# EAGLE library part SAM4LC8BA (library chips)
SAM4L Microcontroller. 64QFN Package. 512 Flash.
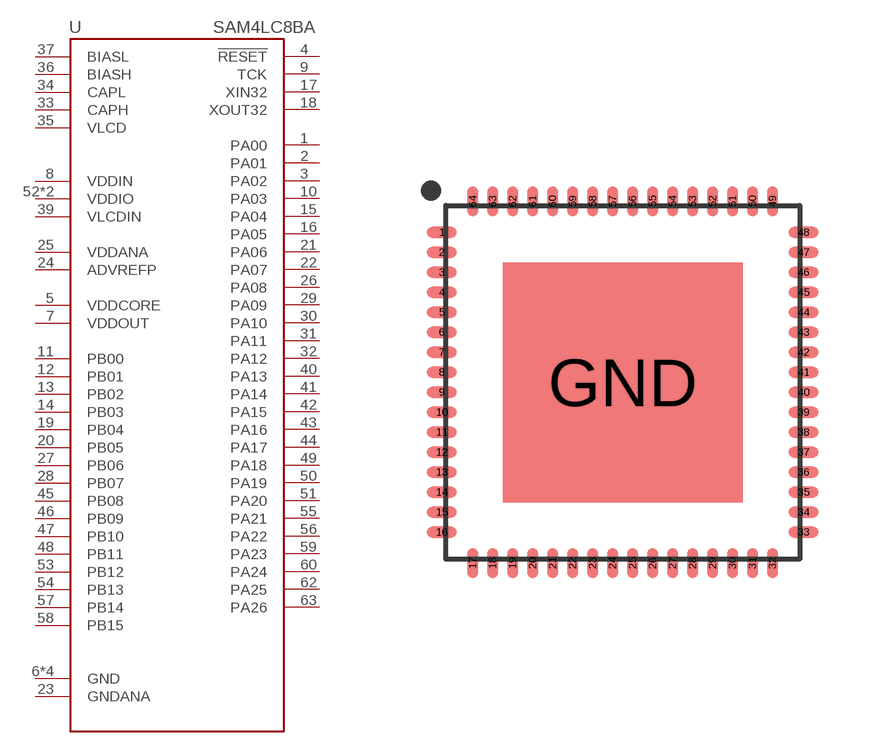
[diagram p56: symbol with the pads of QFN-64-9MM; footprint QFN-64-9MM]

Designator prefix U

## SAM4LC8BA (DIGIKEY: ATSAM4LC8BA-MURCT-ND; MANUFACTURER: Microchip; MPN: ATSAM4LC8BA-MUR)  [QFN-64-9MM]
1  PA00
2  PA01
3  PA02
4  !RESET
5  VDDCORE  pwr
6  GND  pwr
7  VDDOUT  pwr
8  VDDIN  pwr
9  TCK
10  PA03
11  PB00
12  PB01
13  PB02
14  PB03
15  PA04
16  PA05
17  XIN32
18  XOUT32
19  PB04
20  PB05
21  PA06
22  PA07
23  GNDANA  pwr
24  ADVREFP
25  VDDANA  pwr
26  PA08
27  PB06
28  PB07
29  PA09
30  PA10
31  PA11
32  PA12
33  CAPH
34  CAPL
35  VLCD
36  BIASH
37  BIASL
38  GND  pwr
39  VLCDIN  pwr
40  PA13
41  PA14
42  PA15
43  PA16
44  PA17
45  PB08
46  PB09
47  PB10
48  PB11
49  PA18
50  PA19
51  PA20
52  VDDIO  pwr
53  PB12
54  PB13
55  PA21
56  PA22
57  PB14
58  PB15
59  PA23
60  PA24
61  VDDIO  pwr
62  PA25
63  PA26
64  GND  pwr
GND  GND  pwr

## Footprint QFN-64-9MM (pad centres in mm)
smd 0.75 x 0.28: 1 -4.525,3.75; 2 -4.525,3.25; 3 -4.525,2.75; 4 -4.525,2.25; 5 -4.525,1.75; 6 -4.525,1.25; 7 -4.525,0.75; 8 -4.525,0.25; 9 -4.525,-0.25; 10 -4.525,-0.75; 11 -4.525,-1.25; 12 -4.525,-1.75; 13 -4.525,-2.25; 14 -4.525,-2.75; 15 -4.525,-3.25; 16 -4.525,-3.75; 33 4.525,-3.75; 34 4.525,-3.25; 35 4.525,-2.75; 36 4.525,-2.25; 37 4.525,-1.75; 38 4.525,-1.25; 39 4.525,-0.75; 40 4.525,-0.25; 41 4.525,0.25; 42 4.525,0.75; 43 4.525,1.25; 44 4.525,1.75; 45 4.525,2.25; 46 4.525,2.75; 47 4.525,3.25; 48 4.525,3.75
smd 0.28 x 0.75: 17 -3.75,-4.525; 18 -3.25,-4.525; 19 -2.75,-4.525; 20 -2.25,-4.525; 21 -1.75,-4.525; 22 -1.25,-4.525; 23 -0.75,-4.525; 24 -0.25,-4.525; 25 0.25,-4.525; 26 0.75,-4.525; 27 1.25,-4.525; 28 1.75,-4.525; 29 2.25,-4.525; 30 2.75,-4.525; 31 3.25,-4.525; 32 3.75,-4.525; 49 3.75,4.525; 50 3.25,4.525; 51 2.75,4.525; 52 2.25,4.525; 53 1.75,4.525; 54 1.25,4.525; 55 0.75,4.525; 56 0.25,4.525; 57 -0.25,4.525; 58 -0.75,4.525; 59 -1.25,4.525; 60 -1.75,4.525; 61 -2.25,4.525; 62 -2.75,4.525; 63 -3.25,4.525; 64 -3.75,4.525
smd 6 x 6: GND 0,0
